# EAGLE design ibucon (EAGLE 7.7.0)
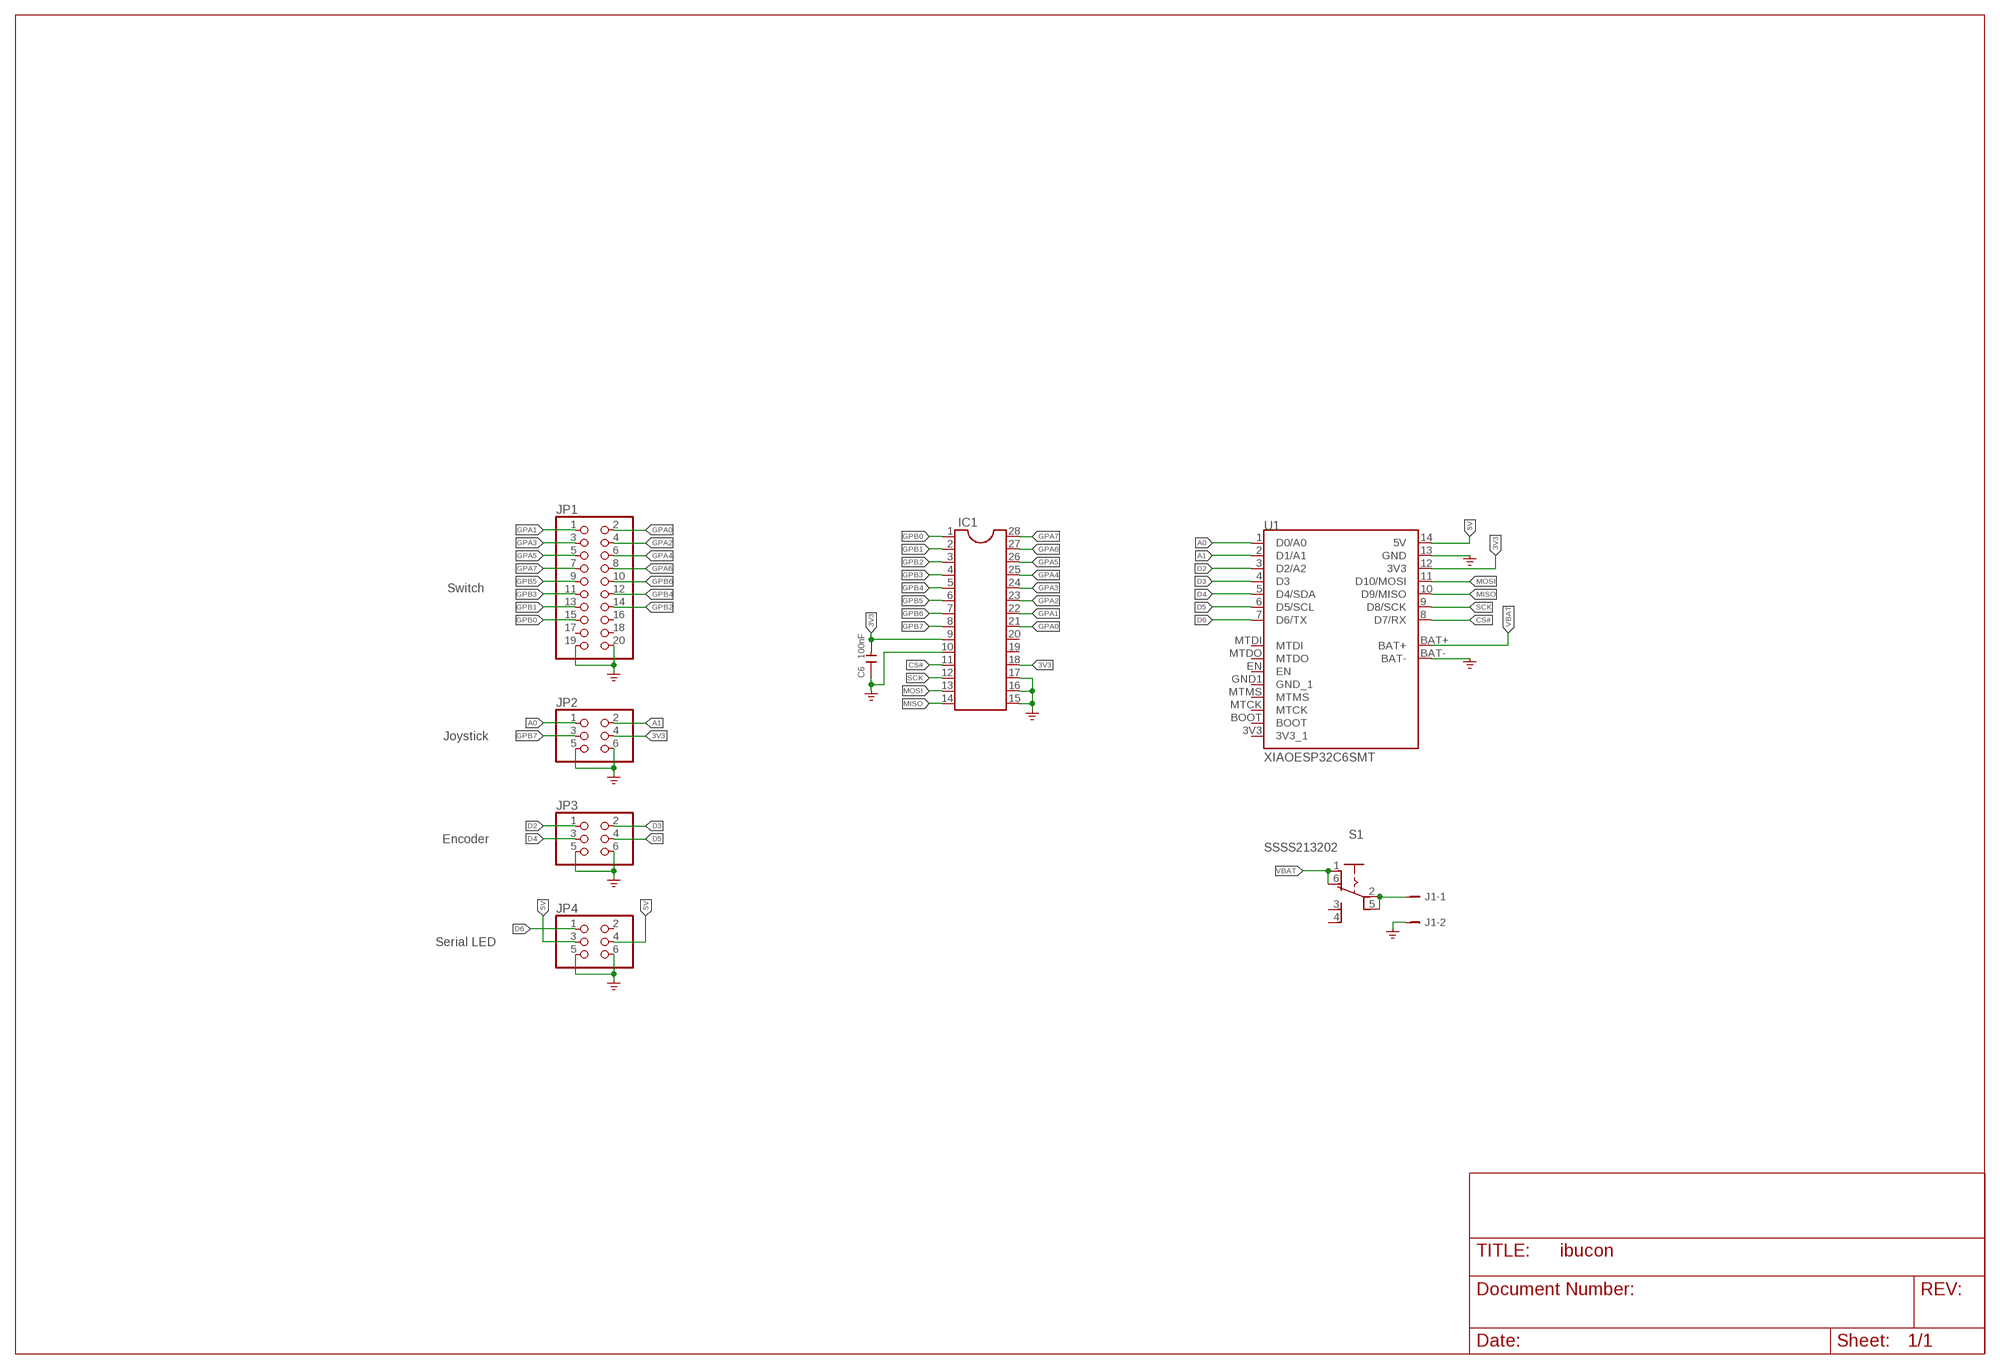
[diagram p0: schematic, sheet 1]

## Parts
C6  100nF  C-0603  [C0603]
IC1  DIL28-3  [DIL28-3]
J1  B2B-PH-K-S  [B2B-PH-K-S]
JP1  PINHD-2X10  [2X10]
JP2  PINHD-2X3  [2X03]
JP3  PINHD-2X3  [2X03]
JP4  PINHD-2X3  [2X03]
S1  SSSS213202  [SSSS213202]
U1  XIAOESP32C6SMT  [XIAOESP32C6-SMT]

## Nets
3V3: C6.2 IC1.9 IC1.18 JP2.4 U1.12(3V3)
5V: JP4.3 JP4.4 U1.14(5V)
A0: JP2.1 U1.1(D0/A0)
A1: JP2.2 U1.2(D1/A1)
CS#: IC1.11 U1.8(D7/RX)
D2: JP3.1 U1.3(D2/A2)
D3: JP3.2 U1.4(D3)
D4: JP3.3 U1.5(D4/SDA)
D5: JP3.4 U1.6(D5/SCL)
D6: JP4.1 U1.7(D6/TX)
GND: C6.1 IC1.10 IC1.15 IC1.16 IC1.17 J1.2 JP1.19 JP1.20 JP2.5 JP2.6 JP3.5 JP3.6 JP4.5 JP4.6 U1.13(GND) U1.BAT- ; supply symbol labelled GND_POWER
GPA0: IC1.21 JP1.2
GPA1: IC1.22 JP1.1
GPA2: IC1.23 JP1.4
GPA3: IC1.24 JP1.3
GPA4: IC1.25 JP1.6
GPA5: IC1.26 JP1.5
GPA6: IC1.27 JP1.8
GPA7: IC1.28 JP1.7
GPB0: IC1.1 JP1.15
GPB1: IC1.2 JP1.13
GPB2: IC1.3 JP1.14
GPB3: IC1.4 JP1.11
GPB4: IC1.5 JP1.12
GPB5: IC1.6 JP1.9
GPB6: IC1.7 JP1.10
GPB7: IC1.8 JP2.3
MISO: IC1.14 U1.10(D9/MISO)
MOSI: IC1.13 U1.11(D10/MOSI)
N$1: J1.1 S1.2(C1) S1.5(C2)
SCK: IC1.12 U1.9(D8/SCK)
VBAT: S1.1(NC1) S1.6(NC2) U1.BAT+
Unconnected: IC1.19 IC1.20 JP1.16 JP1.17 JP1.18 JP4.2 S1.3(NO1) S1.4(NO2) U1.BOOT U1.EN U1.MTCK U1.MTDI U1.MTDO U1.MTMS

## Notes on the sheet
- Switch
- Joystick
- Encoder
- Serial LED

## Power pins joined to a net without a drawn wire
3V3_1: U1.3V3(3V3_1)
GND_1: U1.GND1(GND_1)

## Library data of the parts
C6 = Discrete-small:C*: Ceramic Capacitors
IC1 = ic-package:DIL28: Dual In Line
J1 = con-JST-PH:B2B-PH-K-S: JST-PH 2-way vertical TH; MF: JST; MPN: B2B-PH-K-S
JP1 = pinhead:PINHD-2X10: PIN HEADER
JP2-JP4 = pinhead:PINHD-2X3: PIN HEADER
S1 = matsujirushi:SSSS213202
U1 = matsujirushi:XIAOESP32C6

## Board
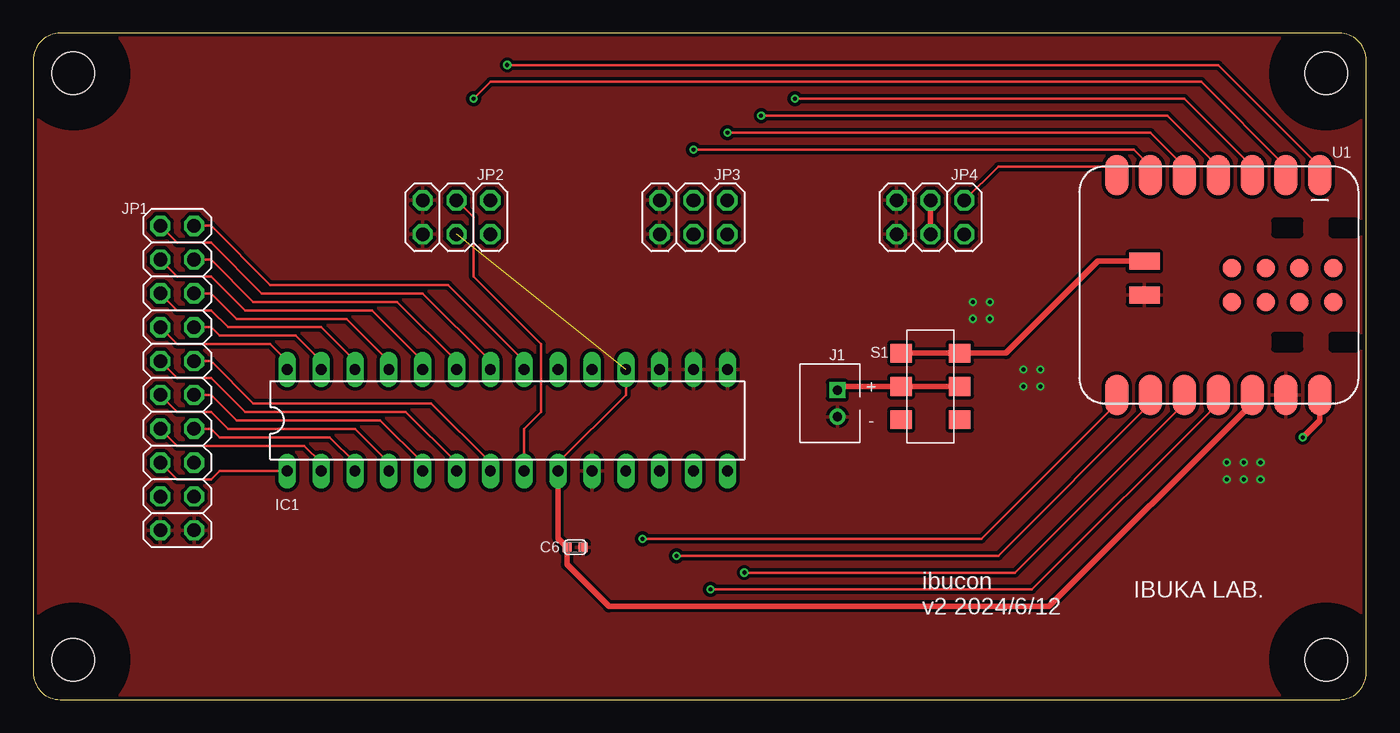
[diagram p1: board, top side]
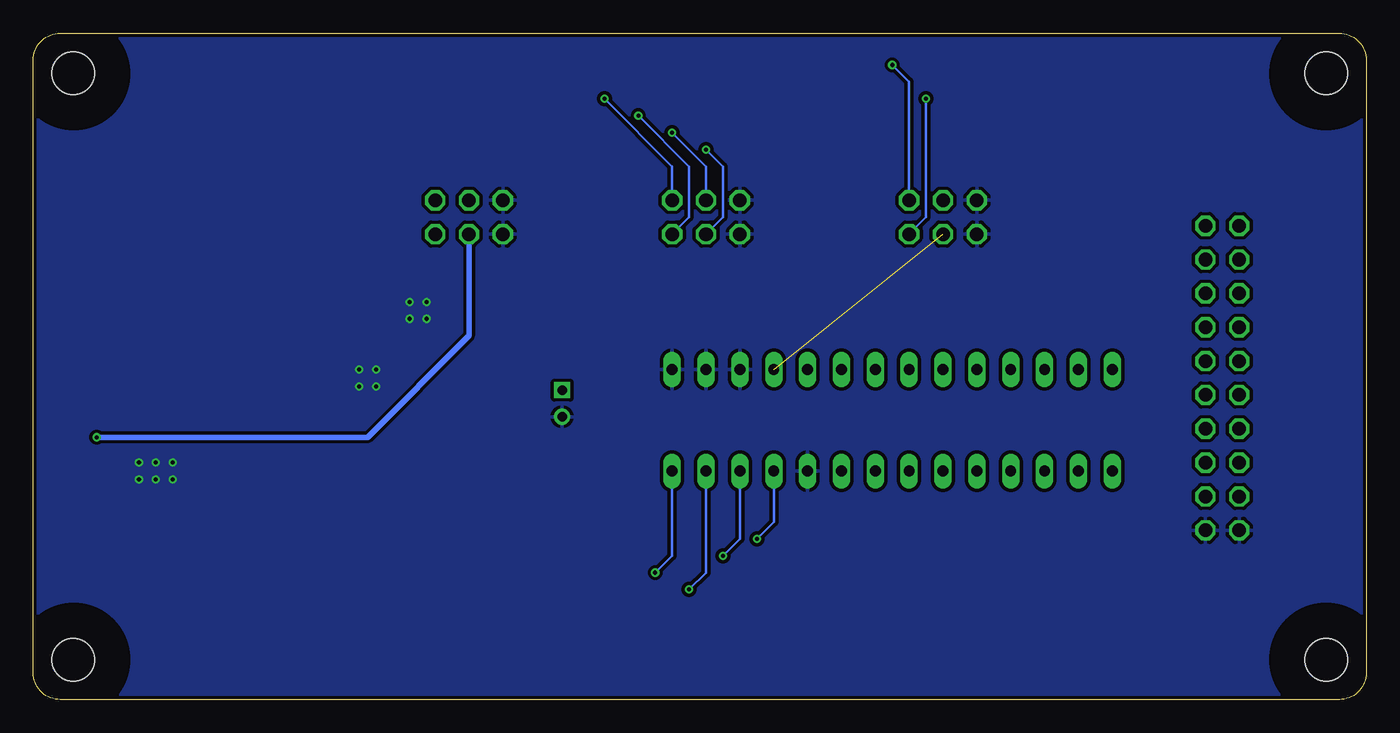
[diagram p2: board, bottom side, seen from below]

Size 100 x 50 mm. Coordinates in mm from the lower left corner, seen from the top.
Outline: 0,48 0,2 arc90 2,0 98,0 arc90 100,2 100,48 arc90 98,50 2,50 arc90 0,48
Copper layers (1*16): Top 0.035mm / dielectric 1.5mm / Bottom 0.035mm
Design rules "SeeedStudio_2layer_DRU_no_angle_20140221": minimum track width 6mil, minimum drill 12mil, track to track 6mil, track to pad 6mil, pad to pad 6mil, via to via 6mil, smd to smd 0mil, copper to edge 10mil, drill to drill 10mil, minimum pad ring 10mil, minimum via ring 6mil, stop-mask expansion 2mil, vias tented up to drill 100mil, thermal gap 10mil
Holes 3.2 mm at 3,3 3,47 97,3 97,47
tRestrict: area -1,-1 to 7,7; area -1,43 to 7,51; area 93,43 to 101,51; area 93,-1 to 101,7
bRestrict: area -1,-1 to 7,7; area -1,43 to 7,51; area 93,43 to 101,51; area 93,-1 to 101,7

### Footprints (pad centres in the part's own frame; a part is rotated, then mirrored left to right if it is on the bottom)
C0603 = smd 0.762 x 0.696: 1 0,0.602; 2 0,-0.602
DIL28-3 = drill 0.813 long: 1 -16.51,-3.81; 2 -13.97,-3.81; 3 -11.43,-3.81; 4 -8.89,-3.81; 5 -6.35,-3.81; 6 -3.81,-3.81; 7 -1.27,-3.81; 8 1.27,-3.81; 9 3.81,-3.81; 10 6.35,-3.81; 11 8.89,-3.81; 12 11.43,-3.81; 13 13.97,-3.81; 14 16.51,-3.81; 15 16.51,3.81; 16 13.97,3.81; 17 11.43,3.81; 18 8.89,3.81; 19 6.35,3.81; 20 3.81,3.81; 21 1.27,3.81; 22 -1.27,3.81; 23 -3.81,3.81; 24 -6.35,3.81; 25 -8.89,3.81; 26 -11.43,3.81; 27 -13.97,3.81; 28 -16.51,3.81
B2B-PH-K-S = drill 0.7 square: 1 1,0 | drill 0.7: 2 -1,0
2X10 = drill 1.016 octagon: 1 -11.43,-1.27; 2 -11.43,1.27; 3 -8.89,-1.27; 4 -8.89,1.27; 5 -6.35,-1.27; 6 -6.35,1.27; 7 -3.81,-1.27; 8 -3.81,1.27; 9 -1.27,-1.27; 10 -1.27,1.27; 11 1.27,-1.27; 12 1.27,1.27; 13 3.81,-1.27; 14 3.81,1.27; 15 6.35,-1.27; 16 6.35,1.27; 17 8.89,-1.27; 18 8.89,1.27; 19 11.43,-1.27; 20 11.43,1.27
2X03 = drill 1.016 octagon: 1 -2.54,-1.27; 2 -2.54,1.27; 3 0,-1.27; 4 0,1.27; 5 2.54,-1.27; 6 2.54,1.27
SSSS213202 = smd 1.4 x 1.6: 1 -2.5,-2.2; 2 0,-2.2; 3 2.5,-2.2; 4 2.5,2.2; 5 0,2.2; 6 -2.5,2.2
XIAOESP32C6-SMT = smd 1.778 x 3.048: 1 7.62,8.255; 2 5.08,8.255; 3 2.54,8.255; 4 0,8.255; 5 -2.54,8.255; 6 -5.08,8.255; 7 -7.62,8.255; 8 -7.62,-8.255; 9 -5.08,-8.255; 10 -2.54,-8.255; 11 0,-8.255; 12 2.54,-8.255; 13 5.08,-8.255; 14 7.62,-8.255 | smd 1.397 x 1.397: 3V3 1.016,-1.27; BOOT 1.016,1.27; EN 6.096,1.27; GND1 6.096,-1.27; MTCK 3.556,-1.27; MTDI 8.636,1.27; MTDO 8.636,-1.27; MTMS 3.556,1.27 | smd 2.286 x 1.27: BAT+ -5.537,1.778; BAT- -5.537,-0.762

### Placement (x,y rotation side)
C6  40.64,11.43 270 top
IC1  35.56,20.95 0 top
J1  60.33,22.23 90 top
JP1  10.79,24.13 270 top
JP2  31.75,36.2 180 top
JP3  49.53,36.2 180 top
JP4  67.31,36.2 180 top
S1  67.31,23.5 270 top
U1  88.9,31.11 0 top

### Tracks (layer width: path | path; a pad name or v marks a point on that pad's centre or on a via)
3V3  (1 unrouted)
  Top 0.203: IC1.9 39.37,17.78 44.45,22.86 IC1.18
  Top 0.406: IC1.9 39.37,12.1 C6.2 40.04,10.13 43.18,6.99 76.2,6.99 91.44,22.23 U1.12
5V  (via drill 0.3)
  Top 0.406: JP4.3 JP4.4 | U1.14 96.52,20.95 v95.25,19.68
  Bottom 0.406: JP4.4 67.31,27.3 74.93,19.68 v95.25,19.68
A0  (via drill 0.3)
  Top 0.203: v35.56,47.62 88.9,47.62 96.52,40.01 U1.1
  Bottom 0.203: JP2.1 34.29,46.35 v35.56,47.62
A1  (via drill 0.3)
  Top 0.203: v33.02,45.09 34.29,46.35 87.63,46.35 93.98,40.01 U1.2
  Bottom 0.203: JP2.2 33.02,36.2 v33.02,45.09
CS#  (via drill 0.3)
  Top 0.203: v45.72,12.06 71.12,12.06 81.28,22.23 U1.8
  Bottom 0.203: v45.72,12.06 44.45,13.34 IC1.11
D2  (via drill 0.3)
  Top 0.203: v57.15,45.09 86.36,45.09 91.44,40.01 U1.3
  Bottom 0.203: JP3.1 52.07,40.01 v57.15,45.09
D3  (via drill 0.3)
  Top 0.203: v54.61,43.81 85.09,43.81 88.9,40.01 U1.4
  Bottom 0.203: JP3.2 50.8,36.2 50.8,40.01 v54.61,43.81
D4  (via drill 0.3)
  Top 0.203: v52.07,42.55 83.82,42.55 86.36,40.01 U1.5
  Bottom 0.203: JP3.3 49.53,40.01 v52.07,42.55
D5  (via drill 0.3)
  Top 0.203: v49.53,41.27 82.55,41.27 83.82,40.01 U1.6
  Bottom 0.203: JP3.4 48.26,36.2 48.26,40.01 v49.53,41.27
D6
  Top 0.203: JP4.1 72.39,40.01 80.64,40.01 U1.7
GND  (via drill 0.3)
  other vias: 92.08,17.78 92.08,16.51 90.81,16.51 90.81,17.78 89.53,17.78 89.53,16.51 75.56,23.5 75.56,24.77 74.3,24.77 74.3,23.5 71.75,28.57 71.75,29.84 70.48,29.84 70.48,28.57
  pour Top (isolate 0.254): 0,50 100,50 100,0 0,0
  pour Bottom (isolate 0.254): 0,50 100,50 100,0 0,0
GPA0
  Top 0.203: JP1.2 13.34,35.56 17.78,31.11 31.11,31.11 36.83,25.4 IC1.21
GPA1
  Top 0.203: JP1.1 10.79,34.29 13.34,34.29 17.14,30.48 29.21,30.48 34.29,25.4 IC1.22
GPA2
  Top 0.203: JP1.4 13.34,33.02 16.51,29.84 27.3,29.84 31.75,25.4 IC1.23
GPA3
  Top 0.203: JP1.3 10.79,31.75 13.34,31.75 15.88,29.21 25.4,29.21 29.21,25.4 IC1.24
GPA4
  Top 0.203: JP1.6 13.34,30.48 15.24,28.57 23.5,28.57 26.67,25.4 IC1.25
GPA5
  Top 0.203: JP1.5 10.79,29.21 13.34,29.21 14.61,27.94 21.59,27.94 24.13,25.4 IC1.26
GPA6
  Top 0.203: JP1.8 13.34,27.94 13.97,27.3 19.68,27.3 21.59,25.4 IC1.27
GPA7
  Top 0.203: JP1.7 10.79,26.67 17.78,26.67 19.05,25.4 IC1.28
GPB0
  Top 0.203: JP1.15 10.79,16.51 13.34,16.51 13.97,17.14 IC1.1
GPB1
  Top 0.203: IC1.2 21.59,17.78 20.32,19.05 10.79,19.05 JP1.13
GPB2
  Top 0.203: IC1.3 24.13,17.78 22.23,19.68 13.97,19.68 13.34,20.32 JP1.14
GPB3
  Top 0.203: JP1.11 10.79,21.59 13.34,21.59 14.61,20.32 24.13,20.32 26.67,17.78 IC1.4
GPB4
  Top 0.203: IC1.5 29.21,17.78 26.04,20.95 15.24,20.95 13.34,22.86 JP1.12
GPB5
  Top 0.203: JP1.9 10.79,24.13 13.34,24.13 15.88,21.59 27.94,21.59 31.75,17.78 IC1.6
GPB6
  Top 0.203: JP1.10 13.34,25.4 16.51,22.23 29.84,22.23 34.29,17.78 IC1.7
GPB7
  Top 0.203: JP2.3 33.02,36.2 33.02,31.75 38.1,26.67 38.1,21.59 36.83,20.32 IC1.8
MISO  (via drill 0.3)
  Top 0.203: v53.34,9.53 73.66,9.53 86.36,22.23 U1.10
  Bottom 0.203: v53.34,9.53 52.07,10.79 IC1.14
MOSI  (via drill 0.3)
  Top 0.203: v50.8,8.26 74.93,8.26 88.9,22.23 U1.11
  Bottom 0.203: v50.8,8.26 49.53,9.53 IC1.13
N$1
  Top 0.406: S1.5 S1.2 60.33,23.5 J1.1
SCK  (via drill 0.3)
  Top 0.203: v48.26,10.79 72.39,10.79 83.82,22.23 U1.9
  Bottom 0.203: v48.26,10.79 46.99,12.06 IC1.12
VBAT
  Top 0.406: S1.1 S1.6 72.98,26 79.88,32.89 U1.BAT+

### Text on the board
tPlace: + | - | ibucon | IBUKA LAB. | v2 2024/6/12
